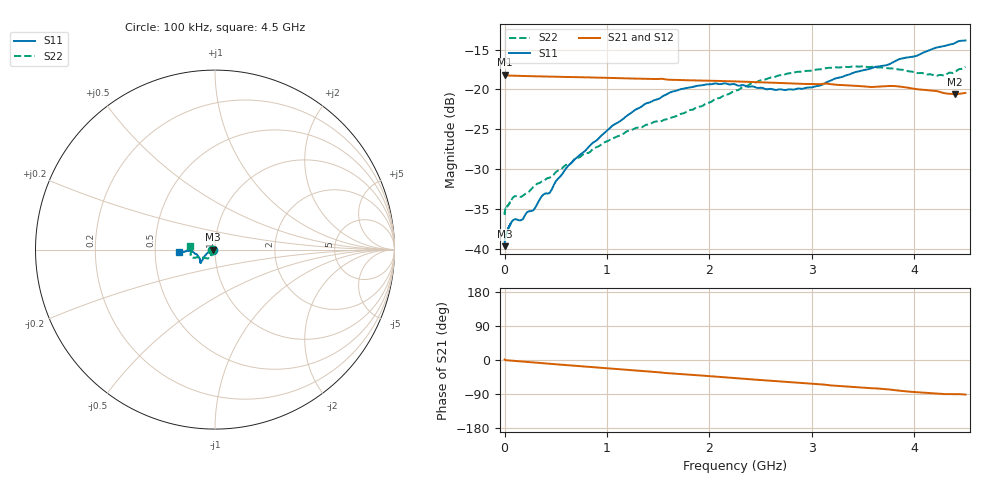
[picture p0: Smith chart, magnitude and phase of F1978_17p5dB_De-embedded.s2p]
! Integrated Device Technology
! Corporate Headquarters
! 6024 Silver Creek Valley Road
! San Jose, CA 95138  USA
! Phone:  1-408-284-8200
! Toll Free:  1-800-223-1366
! Webpage:  http://www.idt.com/
! Timing and RF Division
! 515 Groton Road, Suite 102
! Westford, MA 01886-6024
! Device:  F1978
! Description: 6-bit, 75 ohm, 0.5 dB Digital Step Attenuator
! Frequency:  5.0 MHz -  3.00 GHz
! Package:  4x4 mm QFN Plastic Package: 20 pin
! Ports:  2 RF, 11 DC
!  Pin  1  = D5 (16 dB)
!  Pin  2  = RF1  =  Port 1
!  Pin  3  = Serial Data In (DATA)
!  Pin  4  = Serial Clock (CLK)
!  Pin  5  = Serial Latch Enable (LE)
!  Pin  6  = VDD
!  Pin  7  = NC
!  Pin  8  = NC
!  Pin  9  = NC
!  Pin 10  = GND
!  Pin 11  = GND
!  Pin 12  = NC
!  Pin 13  = VMODE
!  Pin 14  = RF2  =  Port 2
!  Pin 15  = D4 (8 dB)
!  Pin 16  = D3 (4 dB)
!  Pin 17  = D2 (2 dB)
!  Pin 18  = NC
!  Pin 19  = D1 (1 dB)
!  Pin 20  = D0 (0.5 dB)
! State:  35
! Atten State:  17.5 dB
! Voltage:  +3.30 Volts
! Current:  0.561 mA
! Data:  The device was measured on a F1975 evaluation board which has
!  individual transmission lines to the RF pins.  Data was collected
!  using a calibrated network analyzer.  The evaluation board was
!  de-embedded using Automatic Fixture Removal (AFR).
!  The reference plane is the edge of the package pin.
! Misc:
!  Action Tracker AT0416
! Date Measured:  2018-02-08
! Date:  2018-03-26  MJV
! Note:
!  Integrated Device Technology supplies this data as a sample of measured
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# GHz S dB R 75
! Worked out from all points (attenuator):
!   291 points, 100 kHz to 4.5 GHz, reference 75 ohm
!   highest |S21| = -18.17 dB at 100 kHz (marker M1); lowest = -20.6 dB at 4.4 GHz (marker M2)
!   lowest |S11| = -39.7 dB at 100 kHz (marker M3), VSWR 1.02, Z = 73.5 + j0.00591 ohm
!   |S11| at or under -10 dB: start of sweep to end of sweep
!   |S22| runs from -35.8 to -17.1 dB; largest |S21 - S12| = 0.00021
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0.0001  -39.67 179.8  -18.17 1.2  -18.16 1.2  -35.76 -179.0
0.002  -38.79 -177.2  -18.21 0.8  -18.20 0.9  -35.29 -177.4
0.007  -38.40 -176.4  -18.23 0.1  -18.22 0.1  -35.04 -176.3
0.08  -36.42 -170.7  -18.28 -2.1  -18.28 -2.1  -33.59 -165.0
0.16  -36.42 -168.1  -18.31 -3.9  -18.31 -3.9  -33.50 -152.0
0.22  -35.40 -169.6  -18.33 -5.2  -18.33 -5.2  -33.03 -145.6
0.28  -35.19 -168.8  -18.35 -6.5  -18.35 -6.5  -32.25 -142.3
0.36  -33.46 -168.5  -18.37 -8.2  -18.37 -8.3  -31.58 -134.4
0.44  -32.98 -166.4  -18.39 -10.0  -18.39 -10.0  -31.09 -128.6
0.6  -29.91 -163.7  -18.44 -13.4  -18.44 -13.4  -29.47 -123.8
0.76  -27.97 -157.5  -18.48 -16.8  -18.48 -16.8  -28.22 -121.4
1.06  -24.49 -150.5  -18.57 -23.2  -18.57 -23.2  -26.12 -119.7
1.52  -21.09 -140.8  -18.67 -32.7  -18.67 -32.7  -24.03 -128.7
1.88  -19.55 -137.4  -18.88 -40.2  -18.87 -40.1  -22.22 -143.6
2.26  -19.42 -138.8  -19.00 -47.9  -19.00 -47.9  -20.14 -154.8
2.64  -20.06 -148.7  -19.17 -55.7  -19.17 -55.7  -18.43 -158.0
3.02  -19.68 -164.0  -19.33 -63.0  -19.33 -63.0  -17.58 -160.7
3.42  -17.85 -175.0  -19.54 -71.7  -19.54 -71.7  -17.09 -166.6
3.76  -16.83 -176.9  -19.57 -77.9  -19.57 -77.9  -17.36 -173.0
4.2  -14.83 -175.6  -20.19 -88.2  -20.18 -88.2  -18.30 175.5
4.4  -14.18 -174.6  -20.61 -90.2  -20.61 -90.2  -17.84 172.3
4.5  -13.86 -176.4  -20.44 -91.2  -20.44 -91.2  -17.15 170.8
